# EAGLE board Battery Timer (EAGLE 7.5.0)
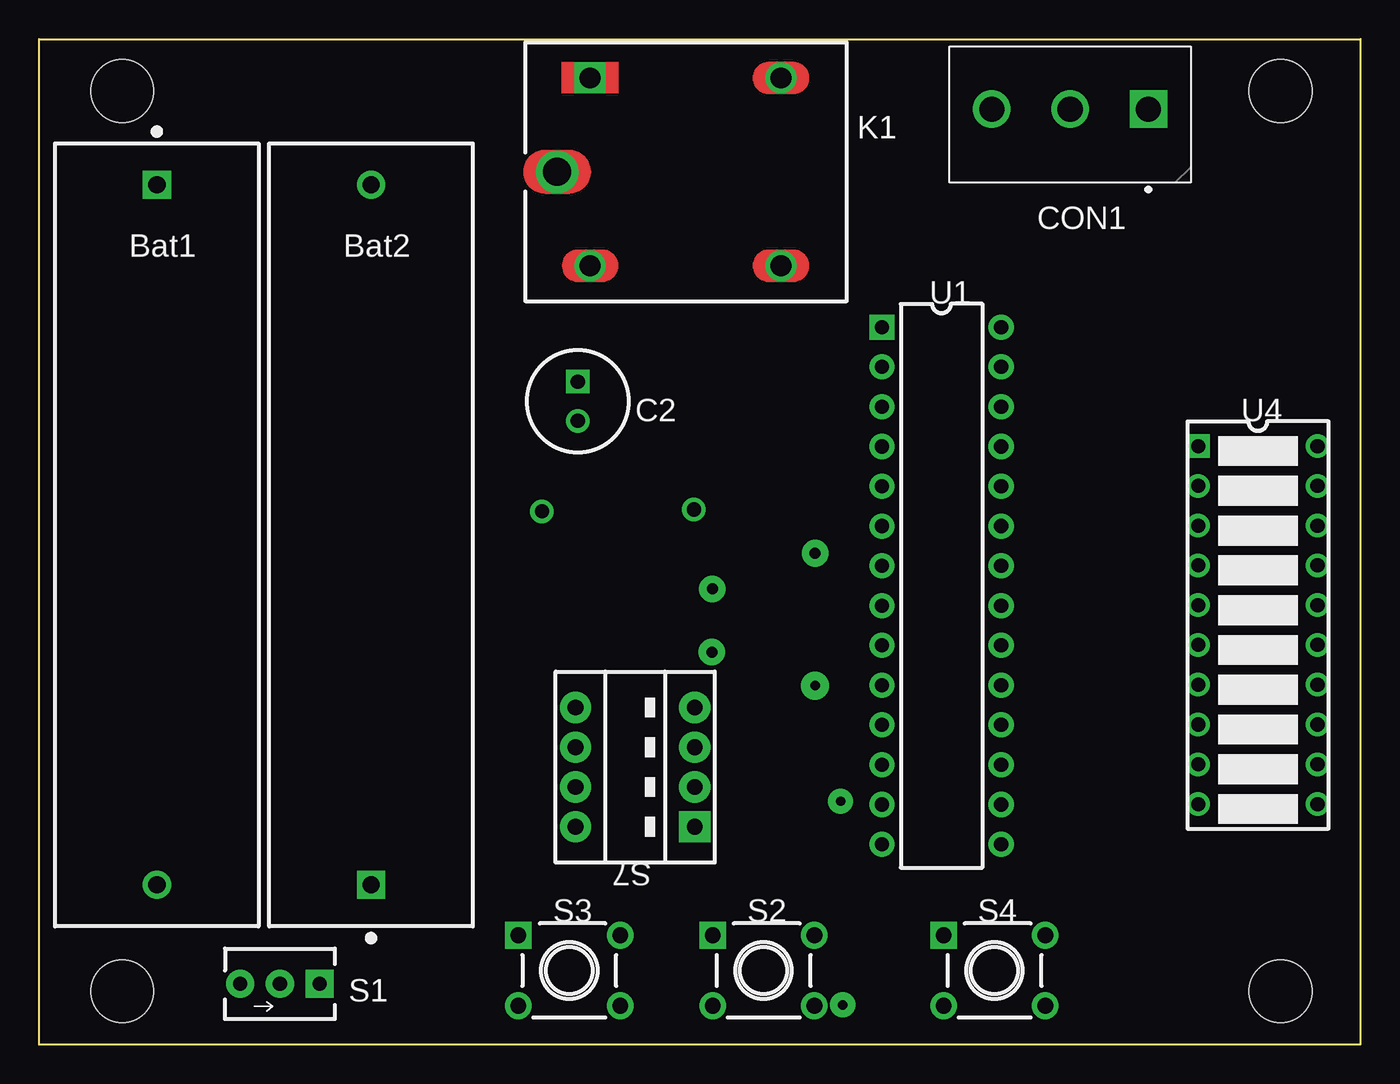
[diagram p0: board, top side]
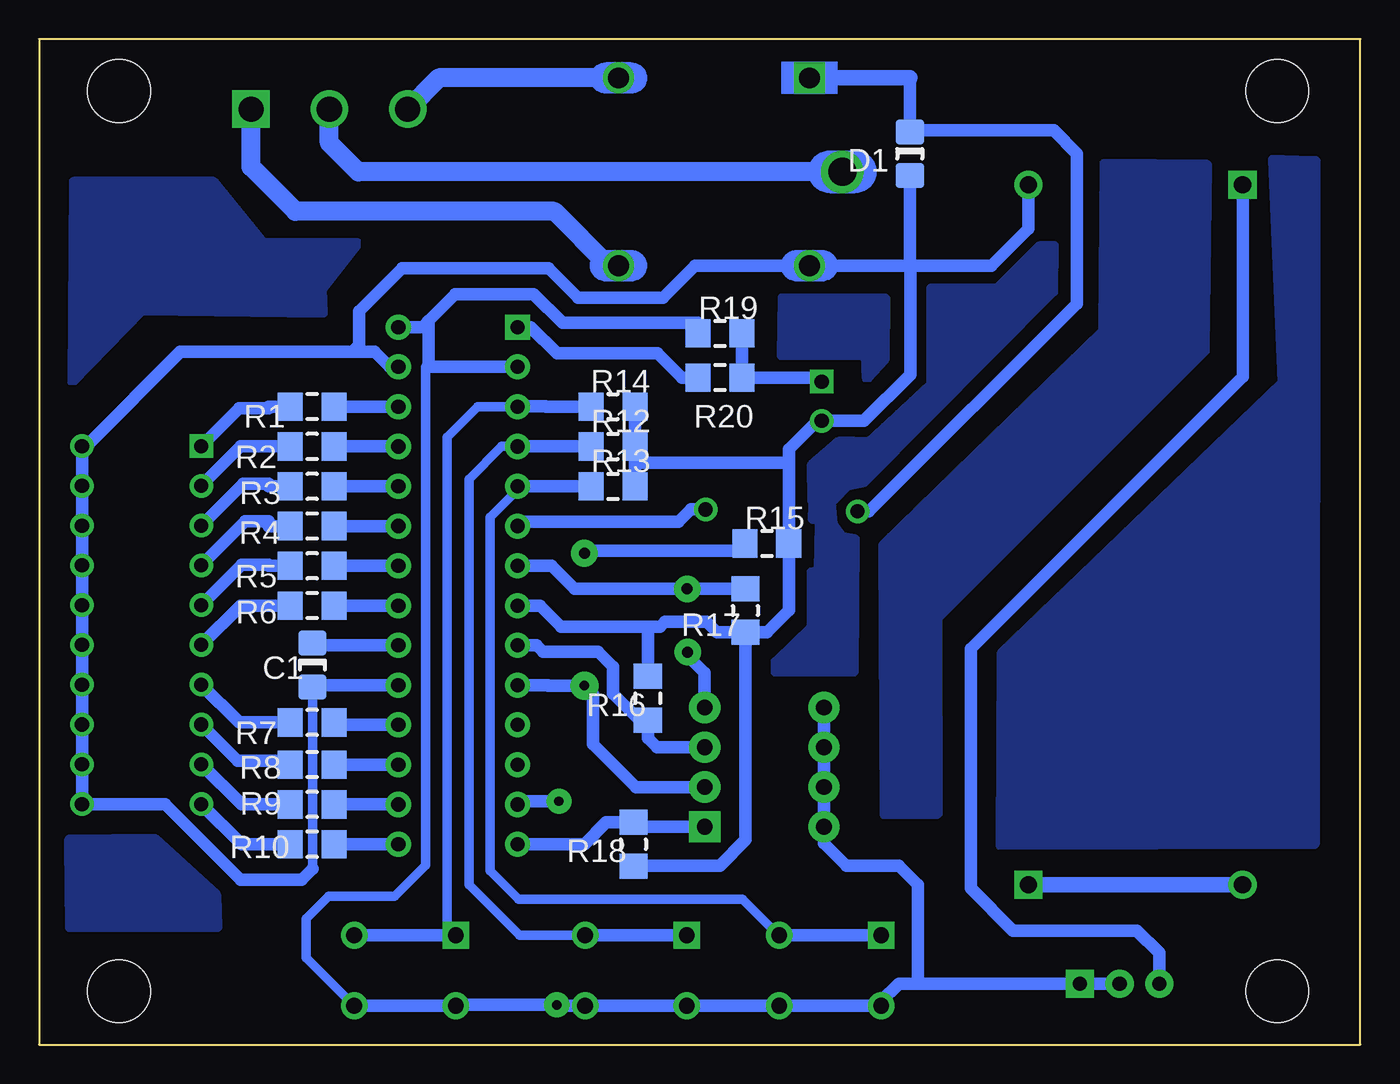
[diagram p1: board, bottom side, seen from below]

Size 84.4 x 64.2 mm. Coordinates in mm from the lower left corner, seen from the top.
Outline: 84.4,64.2 84.4,0 0,0 0,64.2 84.4,64.2
Copper layers (1*16): Top 0.035mm / dielectric 1.5mm / Bottom 0.035mm
Design rules "default *": minimum track width 10mil, minimum drill 0.61mm, track to track 8mil, track to pad 8mil, pad to pad 8mil, via to via 8mil, smd to smd 8mil, copper to edge 40mil, drill to drill 8mil, minimum pad ring 0mil, minimum via ring 8mil, stop-mask expansion 2mil, vias tented up to drill 28mil, thermal gap 10mil
Net classes: 0 Default: width 0.8 mm, clearance 0.33 mm
Holes 4 mm at 79.3,60.89 79.3,3.39 5.3,3.39 5.3,60.89

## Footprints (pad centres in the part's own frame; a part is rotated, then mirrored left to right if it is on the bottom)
2466 = drill 1.1 pad 1.8 square: 1 -22.35,0 | drill 1.1 pad 1.8: 2 22.35,0
2466_Bat2 = drill 1.1 pad 1.8 square: 1 -22.35,0 | drill 1.1 pad 1.8: 2 22.35,0
CAP_1206 = smd 1.6 x 1.8: 1 -1.4,0; 2 1.4,0
CAPR-2.5/6.5h12 = drill 0.9 pad 1.5 square: 1 -1.25,0 | drill 0.9 pad 1.5: 2 1.25,0
SHDRV3W125P500_3X1_1500X830H1240 = drill 1.6 pad 2.4 square: 1 0,0 | drill 1.6 pad 2.4: 2 5,0; 3 10,0
DIO_1206 = smd 1.6 x 1.8: 1 -1.4,0; 2 1.4,0
ZF112 = drill 1.321 pad 1.981 square: 1 -4.861,5.994 | drill 1.321 pad 1.981: 2 -4.861,-5.994; O 7.331,5.994; S 7.331,-5.994 | drill 1.803 pad 2.705: P -6.969,0
Pad = drill 0.9 pad 1.5: 1 0,0
Pad_Pad4 = drill 0.7 pad 1.7: 1 0,0
Pad_Pad5 = drill 0.6 pad 1.8: 1 0,0
RES_1206 = smd 1.6 x 1.8: 1 -1.4,0; 2 1.4,0
RES_1206_R8 = smd 1.6 x 1.8: 1 -1.4,0; 2 1.4,0
RES_1206_R12 = smd 1.6 x 1.8: 1 -1.4,0; 2 1.4,0
RES_1206_R16 = smd 1.6 x 1.8: 1 -1.4,0; 2 1.4,0
RES_1206_R17 = smd 1.6 x 1.8: 1 -1.4,0; 2 1.4,0
RES_1206_R18 = smd 1.6 x 1.8: 1 -1.4,0; 2 1.4,0
RES_1206_R20 = smd 1.6 x 1.8: 1 -1.4,0; 2 1.4,0
CK_GS01MCBE = drill 0.9 pad 1.8 square: 1 -2.54,0 | drill 0.9 pad 1.8: 2 0,0; 3 2.54,0
B3F-1 = drill 1 pad 1.7 square: 1 -3.25,2.25 | drill 1 pad 1.7: 2 3.25,2.25; 3 -3.25,-2.25; 4 3.25,-2.25
BD04 = drill 1 pad 2 square: 1 -3.81,3.81 | drill 1 pad 2: 2 -3.81,1.27; 3 -3.81,-1.27; 4 -3.81,-3.81; 5 3.81,-3.81; 6 3.81,-1.27; 7 3.81,1.27; 8 3.81,3.81
DIP-28 = drill 0.9 pad 1.6 square: 1 -3.81,16.51 | drill 0.9 pad 1.6: 2 -3.81,13.97; 3 -3.81,11.43; 4 -3.81,8.89; 5 -3.81,6.35; 6 -3.81,3.81; 7 -3.81,1.27; 8 -3.81,-1.27; 9 -3.81,-3.81; 10 -3.81,-6.35; 11 -3.81,-8.89; 12 -3.81,-11.43; 13 -3.81,-13.97; 14 -3.81,-16.51; 15 3.81,-16.51; 16 3.81,-13.97; 17 3.81,-11.43; 18 3.81,-8.89; 19 3.81,-6.35; 20 3.81,-3.81; 21 3.81,-1.27; 22 3.81,1.27; 23 3.81,3.81; 24 3.81,6.35; 25 3.81,8.89; 26 3.81,11.43; 27 3.81,13.97; 28 3.81,16.51
10LED_BAR = drill 0.9 pad 1.5 square: 1 -3.81,11.43 | drill 0.9 pad 1.5: 2 -3.81,8.89; 3 -3.81,6.35; 4 -3.81,3.81; 5 -3.81,1.27; 6 -3.81,-1.27; 7 -3.81,-3.81; 8 -3.81,-6.35; 9 -3.81,-8.89; 10 -3.81,-11.43; 11 3.81,-11.43; 12 3.81,-8.89; 13 3.81,-6.35; 14 3.81,-3.81; 15 3.81,-1.27; 16 3.81,1.27; 17 3.81,3.81; 18 3.81,6.35; 19 3.81,8.89; 20 3.81,11.43

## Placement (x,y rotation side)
Bat1  1025  [2466]  7.52,32.54 270 top
Bat2  1025  [2466_Bat2]  21.2,32.54 90 top
C1  47UF  [CAP_1206]  66.95,24.23 270 bottom
C2  47uF  [CAPR-2.5/6.5h12]  34.41,41.08 270 top
CON1  644456-3  [SHDRV3W125P500_3X1_1500X830H1240]  70.86,59.73 180 top
D1  DIODE  [DIO_1206]  28.78,56.88 270 bottom
K1  351  [ZF112]  40.06,55.73 0 top
Pad1  PAD  [Pad]  41.83,34.17 0 top
Pad2  PAD  [Pad]  32.12,34.04 0 top
Pad4  PAD  [Pad_Pad4]  42.97,25.06 0 top
Pad5  PAD  [Pad_Pad5]  49.57,22.91 0 top
Pad6  PAD  [Pad_Pad4]  49.57,31.37 0 top
R1  320  [RES_1206]  66.95,40.73 180 bottom
R2  320  [RES_1206]  66.95,38.19 180 bottom
R3  320  [RES_1206]  66.95,35.65 180 bottom
R4  320  [RES_1206]  66.95,33.11 180 bottom
R5  320  [RES_1206]  66.95,30.57 180 bottom
R6  320  [RES_1206]  66.95,28.03 180 bottom
R7  320  [RES_1206]  66.95,20.57 180 bottom
R8  320  [RES_1206_R8]  66.95,17.87 180 bottom
R9  320  [RES_1206_R8]  66.95,15.33 180 bottom
R10  320  [RES_1206_R8]  66.95,12.79 180 bottom
R12  1K  [RES_1206_R12]  47.74,38.19 0 bottom
R13  1K  [RES_1206_R12]  47.74,35.65 0 bottom
R14  1K  [RES_1206_R12]  47.74,40.73 0 bottom
R15  1K  [RES_1206_R12]  37.92,32 0 bottom
R16  1K  [RES_1206_R16]  45.52,22.11 90 bottom
R17  1K  [RES_1206_R17]  39.28,27.71 270 bottom
R18  1K  [RES_1206_R18]  46.44,12.79 270 bottom
R19  50K  [RES_1206_R12]  40.91,45.42 0 bottom
R20  1K  [RES_1206_R20]  40.91,42.58 180 bottom
S1  JS102011SCQN  [CK_GS01MCBE]  15.38,3.88 180 top
S2  SWITCH_DPST_NO  [B3F-1]  46.27,4.73 0 top
S3  SWITCH_DPST_NO  [B3F-1]  33.87,4.73 0 top
S4  SWITCH_DPST_NO  [B3F-1]  61.02,4.73 0 top
S7  BD04  [BD04]  38.08,17.71 180 top
U1  PIC32MX-D/A 28PINS  [DIP-28]  57.64,29.3 0 top
U4  10LED BAR  [10LED_BAR]  77.85,26.79 0 top

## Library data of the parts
Bat1 Bat2 = common; DATASHEET: http://datasheets.diptrace.com/con_batteries/1025.pdf; MANUFACTURER: Keystone
C1 D1 K1 Pad1 Pad2 Pad4-Pad6 R1-R10 R12-R20 U4 = common
C2 = common; DATASHEET: http://datasheets.diptrace.com/cap/eeefk.pdf; MANUFACTURER: Panasonic
CON1 = common; DATASHEET: http://datasheets.diptrace.com/con_headers/ENG_CD_644456_D2.pdf; MANUFACTURER: TE Connectivity
S1 = common; DATASHEET: http://datasheets.diptrace.com/switches/JS_series.pdf; MANUFACTURER: C&K
S2-S4 = common; DESCRIPTION: Switch; UNTITLED: Normally Open
S7 = common; DATASHEET: http://datasheets.diptrace.com/switches/BD_series.pdf; MANUFACTURER: C&K
U1 = common; MANUFACTURER: MICROMITE

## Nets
Net_0: R1.1 U1.26
Net_1: R2.1 U1.25
Net_2: R3.1 U1.24
Net_3: R4.1 U1.23
Net_4: R5.1 U1.22
Net_5: R6.1 U1.21
Net_6: R10.1 U1.15
Net_7: R9.1 U1.16
Net_8: R8.1 U1.17
Net_9: R7.1 U1.18
Net_10: C1.1 U1.20
Net_11: R18.1 S7.1 U1.14
Net_12: R19.1 S1.2 S2.3 S2.4 S3.3 S3.4 S4.3 S4.4 S7.5 S7.6 S7.7 S7.8 U1.2 U1.13 U1.28
Net_13: R10.2 U4.10
Net_14: R9.2 U4.9
Net_15: Bat2.2 C1.2 C2.2 D1.2 K1.2 R12.2 R13.2 R14.2 R15.2 R16.2 R17.2 R18.2 U1.8 U1.19 U1.27 U4.11 U4.12 U4.13 U4.14 U4.15 U4.16 U4.17 U4.18 U4.19 U4.20
Net_16: R8.2 U4.8
Net_17: R7.2 U4.7
Net_18: R6.2 U4.6
Net_19: R4.2 U4.4
Net_20: R3.2 U4.3
Net_21: R2.2 U4.2
Net_22: R1.2 U4.1
Net_23: Bat1.1 S1.3
Net_24: R12.1 S2.1 S2.2 U1.4
Net_25: R13.1 S3.1 S3.2 U1.5
Net_26: R14.1 S4.1 S4.2 U1.3
Net_27: CON1.1 K1.S
Net_28: Bat1.2 Bat2.1
Net_29: D1.1 K1.1 Pad1.1 Pad2.1 U1.6
Net_30: CON1.2 K1.P
Net_31: CON1.3 K1.O
Net_32: Pad5.1 Pad6.1 R15.1 S7.2 U1.10
Net_33: R5.2 U4.5
Net_34: R20.2 U1.1
Net_35: Pad4.1 R17.1 S7.4 U1.7
Net_36: R16.1 S7.3 U1.9
Net_37: C2.1 R19.2 R20.1

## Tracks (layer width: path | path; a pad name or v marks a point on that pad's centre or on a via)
N$1
  pour Bottom (isolate 0.35, no thermals): 2.88,56.43 2.92,12.8 22.97,12.72 22.9,25.02 4.94,42.3 5.58,56.51 4.94,56.5
N$2
  pour Bottom (isolate 0.35, no thermals): 9.79,56.18 16.37,56.24 16.46,45.54 30.48,31.87 30.4,14.7 27,14.75 27.02,27.22 9.93,44.31 9.93,44.33
N$3
  pour Bottom (isolate 0.35, no thermals): 20.51,50.97 23.21,48.28 27.43,48.28 27.43,42.14 31.4,38.47 33.27,38.52 35.05,36.98 35.02,34.75 33.64,34.79 32.75,35.7 31.68,35.93 19.61,48.1 19.57,50.98
N$4
  pour Bottom (isolate 0.35, no thermals): 32.28,32.26 33.07,32.39 33.69,33.21 33.78,34.28 34.97,34.37 34.99,33.57 34.87,33.57 34.75,33.55 34.64,33.48 34.57,33.37 34.55,33.25 34.63,30.27 35.07,30.13 35.07,26.65 37.38,24.42 37.38,23.81 32.36,23.83
N$5
  pour Bottom (isolate 0.35, no thermals): 64.03,51.16 70.07,51.16 73.26,55.09 82.2,55.09 82.27,42.29 77.82,46.89 66.25,46.73 66.32,48.23
N$6
  pour Bottom (isolate 0.35, no thermals): 30.36,47.65 30.41,43.73 31.52,42.5 31.59,44.01 36.96,44.01 36.88,47.69
N$7
  pour Bottom (isolate 0.35, no thermals): 77.06,13.16 73.09,9.57 73.02,7.49 82.42,7.48 82.47,12.75 82.47,13.1
Net_0
  Bottom 0.8: U1.26 R1.1 | R1.1
Net_1
  Bottom 0.8: U1.25 R2.1 | R2.1
Net_2
  Bottom 0.8: U1.24 R3.1 | R3.1
Net_3
  Bottom 0.8: U1.23 R4.1 | R4.1
Net_4
  Bottom 0.8: U1.22 R5.1 | R5.1
Net_5
  Bottom 0.8: U1.21 R6.1 | R6.1
Net_6
  Bottom 0.8: U1.15 R10.1 | R10.1
Net_7
  Bottom 0.8: U1.16 R9.1 | R9.1
Net_8
  Bottom 0.8: U1.17 R8.1 | R8.1
Net_9
  Bottom 0.8: U1.18 65.55,20.41 R7.1
Net_10
  Bottom 0.8: U1.20 66.81,25.49 C1.1
Net_11
  Bottom 0.8: U1.14 49.57,12.79 48.17,14.19 R18.1 46.16,13.9 S7.1
Net_12  (via drill 0.6 pad 1.6)
  Bottom 0.6: 59.51,43.27 59.7,43.27 59.7,11.45 61.68,9.47 65.91,9.47 67.35,8.03 67.35,5.55 S4.4
  Bottom 0.8: U1.2 59.51,43.27 59.51,46.23 | 59.51,46.23 57.82,47.92 52.81,47.92 50.97,46.08 42.31,46.08 R19.1 | S4.4 S4.3 57.72,2.53 v51.33,2.53 51.33,2.48 S2.4 | S4.4 | S2.3 S2.4 | S2.4 | S3.4 S3.3 30.62,2.75 29.49,3.88 28.26,3.88 | S3.4 | U1.28 59.85,45.81 59.51,46.23 | v51.2,15.53 53.63,15.53 U1.13 | S3.4 S2.3 | S2.3 | S1.2 28.26,3.88 | S7.5 S7.6 | S7.6 | S7.6 S7.7 S7.8 34.27,12.86 32.84,11.43 29.48,11.43 28.26,10.2 28.26,3.88
Net_13
  Bottom 0.8: R10.2 71.47,12.79 U4.10
Net_14
  Bottom 0.8: R9.2 71.47,15.33 U4.9
Net_15
  Bottom 0.6: U1.19 66.27,22.95 66.93,22.29 66.93,11.21
  Bottom 0.8: R16.2 45.52,26.67 | 45.52,26.67 51.05,26.67 52.41,28.03 U1.8 | U1.27 62.02,43.27 62.98,44.22 64.42,44.22 | 64.42,44.22 75.38,44.22 81.28,38.32 81.55,38.32 U4.20 U4.19 U4.18 U4.17 U4.16 U4.15 U4.14 U4.13 U4.12 | U4.12 | U4.12 | U4.12 U4.11 76.35,15.36 71.53,10.53 67.61,10.53 66.93,11.21 | 28.78,49.73 28.75,49.73 28.75,42.78 31.7,39.83 C2.2 34.68,39.83 36.52,38 36.52,37.16 | 28.78,49.73 D1.2 | R17.2 37.92,26.31 36.52,27.72 R15.2 36.52,37.16 | R17.2 39.28,13.06 40.92,11.42 46.4,11.42 R18.2 | 64.42,44.22 63.96,44.68 63.96,46.81 61.21,49.56 51.84,49.56 49.99,47.7 44.53,47.7 42.5,49.73 K1.2 28.78,49.73 | U1.19 66.84,22.95 C1.2 | R17.2 41.11,26.31 41.77,26.98 44.41,26.98 44.73,26.67 45.52,26.67 | R14.2 R12.2 46.34,37.16 | 46.34,37.16 R13.2 | Bat2.2 21.2,52.09 23.56,49.73 28.78,49.73 | 46.34,37.16 36.52,37.16
Net_16
  Bottom 0.8: R8.2 68.6,18.12 71.72,18.12 U4.8
Net_17
  Bottom 0.8: R7.2 | R7.2 71.63,20.57 U4.7
Net_18
  Bottom 0.8: R6.2 71.53,28.03 U4.6
Net_19
  Bottom 0.8: R4.2 69.75,33.11 69.75,33.41 71.22,33.41 U4.4
Net_20
  Bottom 0.8: R3.2 69.75,35.65 69.75,35.8 71.38,35.8 U4.3
Net_21
  Bottom 0.8: R2.2 71.53,38.19 U4.2
Net_22
  Bottom 0.8: R1.2 69.75,40.73 69.75,40.63 71.62,40.63 U4.1
Net_23
  Bottom 0.8: Bat1.1 7.52,42.63 24.88,25.27 24.88,9.97 22.19,7.28 14.27,7.28 12.84,5.85 S1.3
Net_24
  Bottom 0.6: S2.2 53.71,6.98 56.94,10.21 56.94,36.11 54.86,38.19 U1.4
  Bottom 0.8: R12.1 52.82,38.19 | 52.82,38.19 | 52.82,38.19 U1.4 | S2.1 S2.2 | S2.2
Net_25
  Bottom 0.6: U1.5 53.83,35.41 55.59,33.66 55.59,11.11 53.77,9.29 39.46,9.29 37.16,6.98 S3.2
  Bottom 0.8: S3.1 S3.2 | R13.1 U1.5 | U1.5
Net_26
  Bottom 0.6: U1.3 56.39,40.73 58.35,38.76 58.35,6.98 S4.2
  Bottom 0.8: S4.1 S4.2 | S4.2 | U1.3 53.79,40.77 52.04,40.77 52,40.73 R14.1
Net_27
  Bottom 1.2: K1.S 48.02,49.73 51.48,53.2 68.02,53.2 70.86,56.04 CON1.1
Net_28
  Bottom 1: Bat1.2 Bat2.1 | Bat2.1
Net_29
  Bottom 0.8: 28.78,61.72 D1.1 28.69,58.37 19.59,58.37 18.12,56.9 18.12,47.31 31.39,34.04 Pad2.1 | Pad1.1 42.75,34.17 43.55,33.37 53.57,33.37 U1.6
  Bottom 1: 28.78,61.72 K1.1
Net_30
  Bottom 1.2: K1.P 64.01,55.73 65.86,57.57 CON1.2
Net_31
  Bottom 1.2: K1.O 58.87,61.72 CON1.3
Net_32
  Bottom 0.8: R15.1 39.32,31.53 49.56,31.53 Pad6.1 | U1.10 51.88,22.95 51.88,22.91 Pad5.1 49.01,22.36 49.01,19.18 46.28,16.44 S7.2
Net_33
  Bottom 0.8: R5.2 69.75,30.57 69.75,30.65 71.45,30.65 U4.5
Net_34
  Bottom 0.8: U1.1 52.99,45.81 51.32,44.14 44.89,44.14 43.33,42.58 R20.2
Net_35  (via drill 0.7 pad 1.7)
  Bottom 0.8: R17.1 43,29.11 | 43,29.11 50.2,29.11 51.65,30.57 U1.7 | S7.4 41.89,23.74 42.97,24.83 Pad4.1 | v43,29.09 43,29.11
Net_36
  Bottom 0.8: U1.9 52.61,25.49 52.19,25.07 48.69,25.07 47.75,24.13 47.75,22.4 46.06,20.71 R16.1 45.52,19.56 44.94,18.98 S7.3
Net_37
  Bottom 0.8: C2.1 34.66,42.58 R20.1 R19.2

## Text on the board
tPlace: K1 | CON1 | Bat1 | Bat2 | U1 | C2 | U4 | S7 | S3 | S2 | S4 | S1
bPlace: D1 | R19 | R14 | R20 | R12 | R1 | R13 | R2 | R3 | R15 | R4 | R5 | R17 | R6 | C1 | R16 | R7 | R8 | R9 | R18 | R10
